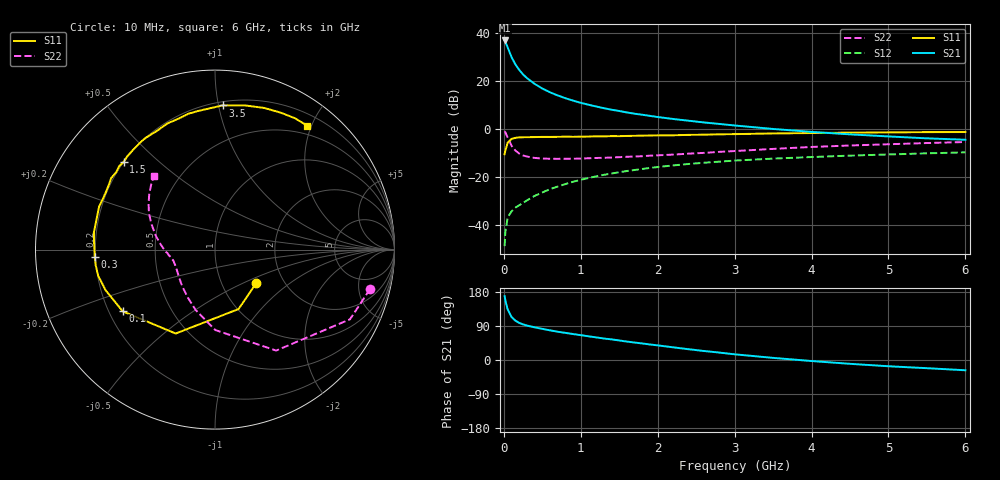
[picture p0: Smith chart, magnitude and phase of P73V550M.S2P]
! SIEMENS Small Signal Semiconductors
! BFP196
! Si NPN RF Bipolar Junction Transistor in SOT143
! VCE = 3.5 V  IC = 50 mA
! Common Emitter S-Parameters:  May  1996
# GHz  S  MA  R  50
!  f  S11  S21  S12  S22
! GHz  MAG  ANG  MAG  ANG  MAG  ANG  MAG  ANG
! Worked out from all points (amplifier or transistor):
!   36 points, 10 MHz to 6 GHz, reference 50 ohm
!   highest |S21| = 36.9 dB at 10 MHz (marker M1)
!   |S21| within 3 dB of that: start of sweep to 51.06 MHz
!   unconditionally stable (mu >= 1): 452.4 MHz to 4.193 GHz
!   at 250 MHz: K = 0.84, MSG = 26.8 dB, |S12| = -30.8 dB
!   at 1.4 GHz: K = 1.08, MAG = 11.5 dB, |S12| = -18.6 dB
!   at 6 GHz: K = 0.97, MSG = 2.6 dB, |S12| = -9.8 dB
!   S11 on the Smith chart (normalised r, x): 10 MHz: 1.45, -0.60; 100 MHz: 0.26, -0.29; 300 MHz: 0.20, -0.03; 1.5 GHz: 0.20, +0.39; 3.5 GHz: 0.23, +1.03; 6 GHz: 0.36, +1.94
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0.01  0.2964 -39.3  69.7 168.5  0.0036 81.4  0.8915 -14.3
0.02  0.3563 -68.4  65.33 156.9  0.0072 72.5  0.8464 -27.3
0.05  0.5163 -115.1  49.83 133.3  0.0142 55.4  0.6577 -58.8
0.1  0.6187 -146.2  31.36 113.6  0.0192 49.3  0.4481 -89.8
0.15  0.6504 -159.7  22.16 103.8  0.0228 49.7  0.3536 -107.7
0.2  0.6669 -167.4  16.99 97.9  0.0257 52.0  0.3064 -119.8
0.25  0.6705 -172.6  13.65 93.9  0.0287 54.4  0.2793 -129.2
0.3  0.6712 -176.6  11.46 90.9  0.0324 56.6  0.2655 -135.5
0.4  0.6752 176.3  8.687 86.2  0.0401 59.2  0.2485 -145.2
0.5  0.6818 172.0  6.945 82.2  0.0474 61.6  0.2413 -151.5
0.6  0.6806 167.4  5.796 78.3  0.0556 62.0  0.2387 -155.9
0.7  0.6837 163.1  4.985 74.6  0.063 62.4  0.238 -159.0
0.8  0.6887 159.6  4.366 71.6  0.0708 62.0  0.239 -161.7
0.9  0.6854 155.8  3.883 68.5  0.0792 61.4  0.239 -164.0
1.1  0.6924 148.8  3.193 62.5  0.0947 60.0  0.2447 -167.4
1.5  0.7056 136.1  2.364 51.6  0.1252 55.2  0.2578 -172.6
2.2  0.7361 116.2  1.61 33.5  0.1733 45.3  0.2914 177.7
2.8  0.7714 101.0  1.269 19.6  0.2078 36.5  0.3322 168.2
3.5  0.8045 87.0  0.997 5.6  0.2405 26.6  0.3832 157.8
4.5  0.8356 70.8  0.77 -10.1  0.2775 14.7  0.4511 145.1
5.5  0.8568 58.7  0.636 -21.6  0.3098 4.0  0.5078 134.5
6  0.8606 53.3  0.594 -27.1  0.3242 -1.8  0.5332 129.4
